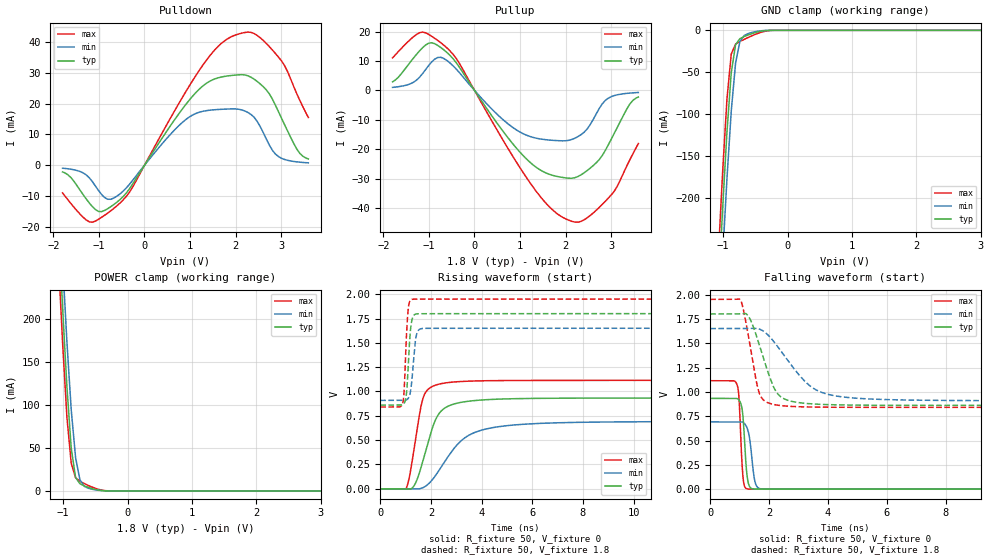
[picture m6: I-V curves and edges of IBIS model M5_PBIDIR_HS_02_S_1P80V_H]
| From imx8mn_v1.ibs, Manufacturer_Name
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[Model] M5_PBIDIR_HS_02_S_1P80V_H
Model_type I/O
Vinl  =  0.54
Vinh  =  1.26
Vmeas =  0.9
| Capacitance   typ   min   max
C_comp   1.4062710684e-12   1.31845087786e-12   1.45127599534e-12
| Variables   typ   min   max
[GND Clamp Reference]   0   0   0
[POWER Clamp Reference]   1.8   1.65   1.95
[Pulldown Reference]   0   0   0
[Pullup Reference]   1.8   1.65   1.95
[Temperature Range]   25   125   -40
[Voltage Range]   1.8   1.65   1.95
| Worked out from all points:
|   slope of the pulldown table from 0 to 0.27 V, typ, clamps not added: 43.7 ohm
|   slope of the pullup table from 0 to 0.27 V, typ, clamps not added: 43.6 ohm
|   GND clamp passes 1 mA (typ) near -0.41 V on its own axis
|   POWER clamp passes 1 mA (typ) near -0.45 V on its own axis
|   falling waveform, R_fixture 50, V_fixture 0: 20-80 % time 122ps typ, 163ps min, 101ps max; typ from 0.933 V to 0 V
|   falling waveform, R_fixture 50, V_fixture 1.8: 20-80 % time 626ps typ, 1.21ns min, 395ps max; typ from 1.8 V to 0.86 V
|   rising waveform, R_fixture 50, V_fixture 0: 20-80 % time 682ps typ, 1.33ns min, 425ps max; typ from 0 V to 0.933 V
|   rising waveform, R_fixture 50, V_fixture 1.8: 20-80 % time 128ps typ, 155ps min, 113ps max; typ from 0.86 V to 1.8 V
[GND Clamp]
| Voltage   I(typ)   I(min)   I(max)
-1.8V     -1.55A     -1.599A    -1.507A
-1.076V   -314.9mA   -373.7mA   -269.5mA
-1.009V   -213.2mA   -272mA     -169.8mA
-941.4mV  -121.7mA   -177.5mA   -82.37mA
-874.1mV  -50.6mA    -96.19mA   -28.29mA
-806.9mV  -17.14mA   -38.88mA   -16.37mA
-739.7mV  -9.899mA   -13.25mA   -13.3mA
-672.4mV  -7.363mA   -6.1mA     -10.74mA
-605.2mV  -5.351mA   -3.675mA   -8.301mA
-470.7mV  -2.028mA   -1.167mA   -3.928mA
-269mV    -32.97uA   -24.73uA   -158.8uA
3.6V      0A         0A         0A
[POWER Clamp]
| Voltage   I(typ)   I(min)   I(max)
-1.8V     1.551A     1.591A     1.512A
-1.076V   314.9mA    367.7mA    272mA
-1.009V   213mA      266.5mA    172.2mA
-941.4mV  120.9mA    173.2mA    85.48mA
-874.1mV  49.37mA    93.93mA    31.94mA
-806.9mV  15.67mA    38.77mA    15.36mA
-739.7mV  8.383mA    12.98mA    11.23mA
-672.4mV  5.889mA    5.395mA    8.598mA
-605.2mV  4.004mA    3.004mA    6.202mA
-470.7mV  1.209mA    899.6uA    2.273mA
-269mV    8.867uA    21.52uA    34.39uA
3.6V      0A         0A         0A
[Pulldown]
| Voltage   I(typ)   I(min)   I(max)
-1.8V     -2.147mA   -951.2uA   -8.956mA
-1.21V    -12.26mA   -4.099mA   -18.34mA
-806.9mV  -14.06mA   -11.02mA   -15.48mA
-537.9mV  -11.11mA   -9.274mA   -12.24mA
931mV     20.14mA    15.09mA    24.42mA
1.552V    28.03mA    18.01mA    37.52mA
2.069V    29.32mA    18.17mA    42.56mA
2.405V    27.96mA    15.61mA    42.73mA
2.607V    25.51mA    10.67mA    40.5mA
2.943V    17.4mA     2.828mA    35.09mA
3.347V    5.257mA    1.104mA    23.19mA
3.6V      2.032mA    786.8uA    15.48mA
[Pullup]
| Voltage   I(typ)   I(min)   I(max)
-1.8V     2.895mA    1.013mA    11.04mA
-1.21V    13.37mA    4.412mA    19.59mA
-874.1mV  15.87mA    10.62mA    17.7mA
-403.4mV  9.449mA    7.287mA    10.9mA
496.6mV   -11.17mA   -8.121mA   -13.5mA
1.117V    -22.95mA   -15.08mA   -29.1mA
1.676V    -28.71mA   -16.94mA   -40.09mA
2.136V    -29.9mA    -16.72mA   -44.54mA
2.674V    -24.66mA   -8.033mA   -40.8mA
3.01V     -16.45mA   -2.11mA    -35.46mA
3.414V    -4.625mA   -928.3uA   -23.61mA
3.6V      -2.257mA   -731.5uA   -18.09mA
[Ramp]
dV/dt_r   0.559581/0.6818n  0.41457/1.32883n  0.668538/0.42482n
dV/dt_f   0.563767/0.625631n  0.444874/1.21182n  0.665669/0.394516n
R_load = 50
[Falling Waveform]
R_fixture = 50
V_fixture = 0
V_fixture_min = 0
V_fixture_max = 0
| Time   V(typ)   V(min)   V(max)
0s        932.6mV    691mV      1.114V
909.8ps   931.1mV    691mV      1.073V
977.1ps   915mV      690.9mV    931.9mV
1.065ns   848.8mV    690.6mV    335.7mV
1.124ns   695.8mV    683.7mV    88.67mV
1.245ns   150.1mV    632.6mV    3.743mV
1.383ns   9.309mV    407.7mV    672.3uV
1.56ns    786.8uV    39.76mV    460.8uV
2.041ns   335.9uV    514.3uV    270uV
333.3ns   124.3nV    586.1nV    100.3nV
[Falling Waveform]
R_fixture = 50
V_fixture = 1.8
V_fixture_min = 1.65
V_fixture_max = 1.95
| Time   V(typ)   V(min)   V(max)
0s        1.8V       1.65V      1.95V
1.036ns   1.802V     1.65V      1.94V
1.352ns   1.747V     1.652V     1.474V
1.609ns   1.536V     1.65V      1.045V
1.794ns   1.359V     1.626V     920mV
2.361ns   957.6mV    1.435V     859.9mV
3.624ns   873.3mV    1.016V     843mV
5.307ns   862.5mV    928.2mV    840.8mV
10.62ns   860.4mV    909.1mV    840.5mV
333.3ns   860.4mV    908.5mV    840.6mV
[Rising Waveform]
R_fixture = 50
V_fixture = 0
V_fixture_min = 0
V_fixture_max = 0
| Time   V(typ)   V(min)   V(max)
0s        91.69nV    585.2nV    87.91nV
1.031ns   -1.943mV   -598.8uV   9.459mV
1.329ns   29.69mV    -2.311mV   397.2mV
1.62ns    229.2mV    5.248mV    862.9mV
1.887ns   477.6mV    46.87mV    1.022V
2.202ns   721.2mV    144.4mV    1.067V
2.546ns   829.8mV    280.7mV    1.087V
3.328ns   894.6mV    522.2mV    1.104V
4.404ns   918.7mV    627mV      1.111V
333.3ns   932.6mV    691mV      1.114V
[Rising Waveform]
R_fixture = 50
V_fixture = 1.8
V_fixture_min = 1.65
V_fixture_max = 1.95
| Time   V(typ)   V(min)   V(max)
0s        860.4mV    908.5mV    840.6mV
878.8ps   863.5mV    908.5mV    876.2mV
943.3ps   878.6mV    908.4mV    1.019V
1.019ns   946.1mV    911.6mV    1.494V
1.106ns   1.271V     930.9mV    1.856V
1.215ns   1.685V     1.04V      1.943V
1.381ns   1.794V     1.508V     1.949V
1.548ns   1.799V     1.639V     1.949V
2.31ns    1.8V       1.65V      1.95V
333.3ns   1.8V       1.65V      1.95V
[Add Submodel]
| Submodel Name Mode
M5_PBIDIR_HS_02_S_1P80V_T_H All
